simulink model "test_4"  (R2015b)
settings: Solver=VariableStepAuto  StartTime=0.0  StopTime=10  RelTol=1e-3
undefined symbols (not defined in the file or in its folder): fir1
libraries: dsparch4 x1

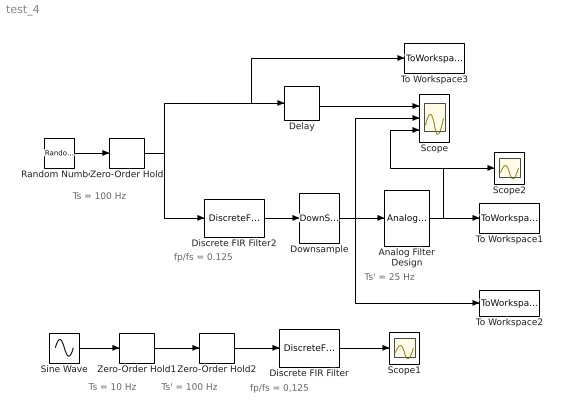
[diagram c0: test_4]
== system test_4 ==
  note: fp/fs = 0.125
  note: fp/fs = 0,125
  note: Ts' = 100 Hz
  note: Ts = 10 Hz
  note: Ts' = 25 Hz
  note: Ts = 100 Hz
  Analog Filter Design : dsparch4/Analog Filter Design  method=Butterworth  filttype=Lowpass  N=8  Wlo=2*pi*5  Whi=80  Rp=2  Rs=40
  Delay : Delay  DelayLength=64
  Discrete FIR Filter : DiscreteFir  Coefficients=fir1(128,0.025)
  Discrete FIR Filter2 : DiscreteFir  Coefficients=fir1(128,0.25)
  Downsample : DownSample  N=4  RateOptions=Allow multirate processing
  Random Number : RandomNumber  SampleTime=0
  Scope : Scope  NumInputPorts=3
  Scope1 : Scope
  Scope2 : Scope
  Sine Wave : Sin  Frequency=2*pi*1  SampleTime=0
  To Workspace1 : ToWorkspace  VariableName=y2  SaveFormat=Timeseries  SampleTime=-1
  To Workspace2 : ToWorkspace  VariableName=y3  SaveFormat=Timeseries  SampleTime=-1
  To Workspace3 : ToWorkspace  VariableName=y1  SaveFormat=Timeseries  SampleTime=-1
  Zero-Order Hold : ZeroOrderHold  SampleTime=0.01
  Zero-Order Hold1 : ZeroOrderHold  SampleTime=0.1
  Zero-Order Hold2 : ZeroOrderHold  SampleTime=0.01
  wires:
  Random Number/1 -> Zero-Order Hold/1
  Zero-Order Hold/1 -> Delay/1, To Workspace3/1, Discrete FIR Filter2/1
  Discrete FIR Filter/1 -> Scope1/1
  Downsample/1 -> To Workspace2/1, Analog Filter Design/1, Scope/2
  Zero-Order Hold1/1 -> Zero-Order Hold2/1
  Analog Filter Design/1 -> Scope2/1, Scope/3, To Workspace1/1
  Zero-Order Hold2/1 -> Discrete FIR Filter/1
  Sine Wave/1 -> Zero-Order Hold1/1
  Delay/1 -> Scope/1
  Discrete FIR Filter2/1 -> Downsample/1
